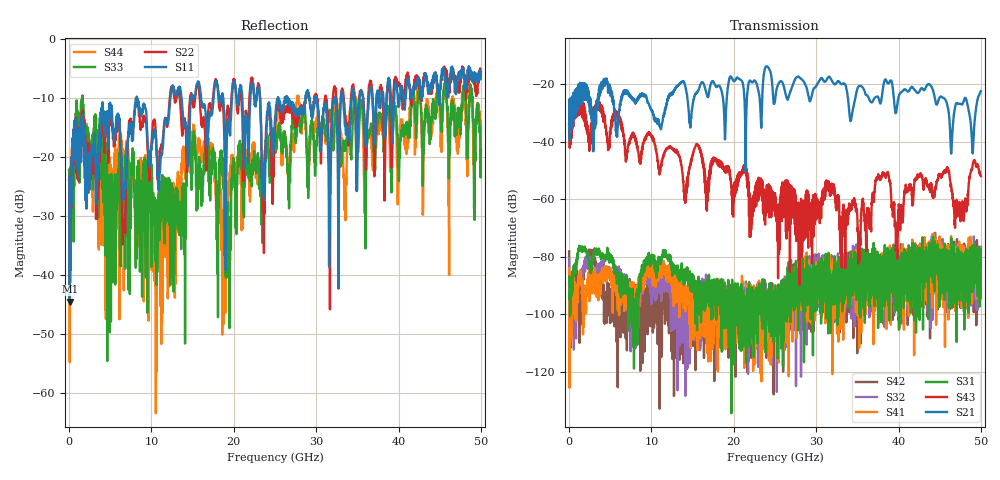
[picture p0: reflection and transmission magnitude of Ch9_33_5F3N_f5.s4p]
!Agilent Technologies,N5247A,US51170199,A.09.90.13
!Agilent N5247A: A.09.90.13
!Date: Wednesday, December 16, 2015 12:08:20
!Correction: S11(Full 4 Port(1,2,3,4))
!S12(Full 4 Port(1,2,3,4))
!S13(Full 4 Port(1,2,3,4))
!S14(Full 4 Port(1,2,3,4))
!S21(Full 4 Port(1,2,3,4))
!S22(Full 4 Port(1,2,3,4))
!S23(Full 4 Port(1,2,3,4))
!S24(Full 4 Port(1,2,3,4))
!S31(Full 4 Port(1,2,3,4))
!S32(Full 4 Port(1,2,3,4))
!S33(Full 4 Port(1,2,3,4))
!S34(Full 4 Port(1,2,3,4))
!S41(Full 4 Port(1,2,3,4))
!S42(Full 4 Port(1,2,3,4))
!S43(Full 4 Port(1,2,3,4))
!S44(Full 4 Port(1,2,3,4))
!S4P File: Measurements: <S11,S12,S13,S14>,
!<S21,S22,S23,S24>,
!<S31,S32,S33,S34>,
!<S41,S42,S43,S44>:
# Hz S  dB  R 50
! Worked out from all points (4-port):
!   3201 points, 10 MHz to 50 GHz, reference 50 ohm
!   strongest paths, dB at 10 MHz, 12.51 GHz, 25 GHz, 37.5 GHz, 50 GHz:
!     S21: -34.5, -23.5, -25.9, -24.4, -22.5
!     S43: -34.6, -42.5, -58.0, -52.2, -52.0
!     S31: -89.5, -83.7, -95.7, -81.7, -83.5
!     S41: -84.0, -85.6, -96.7, -84.9, -93.6
!     S32: -80.7, -93.5, -95.7, -90.1, -76.6
!     S42: -78.2, -92.7, -98.1, -89.5, -77.0
!   lowest |S11| = -44.5 dB at 88.11 MHz (marker M1), VSWR 1.01, Z = 50.4 + j0.485 ohm
!   |S11| at or under -10 dB: start of sweep to 8.131 GHz; 8.251 GHz to 12.28 GHz (4.032 GHz wide, 39.3 % of centre); 23.19 GHz to 25.35 GHz (2.16 GHz wide, 8.9 % of centre)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
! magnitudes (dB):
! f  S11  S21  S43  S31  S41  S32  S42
! 10 MHz  -23.7  -34.5  -34.6  -89.5  -84.0  -80.7  -78.2
! 88.11 MHz  -44.5  -39.6  -42.2  -94.9  -90.5  -106.5  -100.1
! 10.49 GHz  -15.9  -32.9  -41.9  -82.8  -87.5  -91.1  -91.0
! 15.07 GHz  -9.7  -26.4  -44.0  -87.6  -104.5  -95.6  -111.1
! 18.76 GHz  -10.5  -26.6  -49.1  -96.3  -101.6  -96.8  -107.0
! 35.24 GHz  -10.6  -20.6  -76.2  -100.0  -92.7  -85.1  -93.7
! 50 GHz  -5.7  -22.5  -52.0  -83.5  -93.6  -76.6  -77.0
